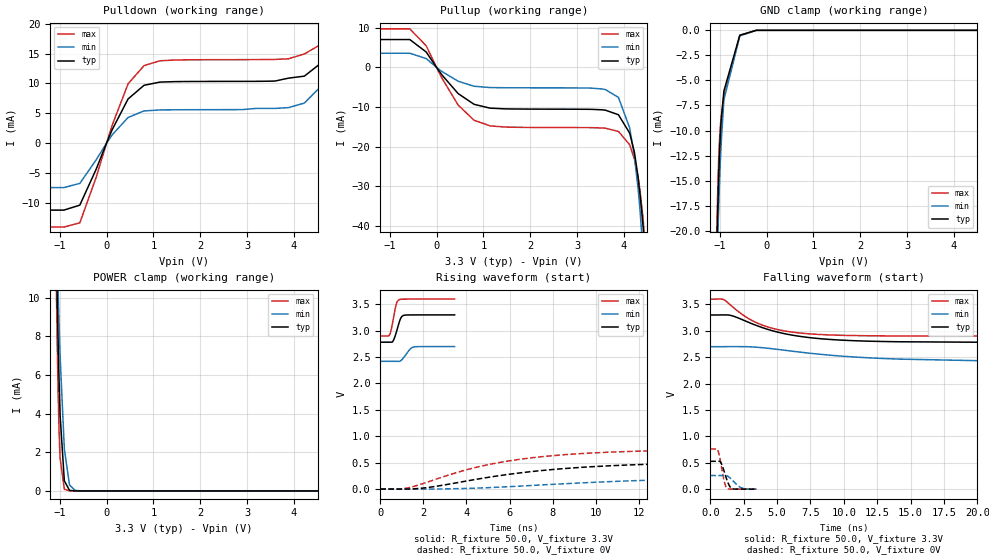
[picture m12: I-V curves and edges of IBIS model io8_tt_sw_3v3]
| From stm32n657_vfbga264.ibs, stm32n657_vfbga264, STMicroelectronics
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[Model]   io8_tt_sw_3v3
Model_type I/O
Polarity   Non-Inverting
Enable   Active-Low
| CAP_THRESHOLD on pad IOTT is "UDTCAPC" :
| Rising=30.0% of vddiov33sw   Falling=70.0% of vddiov33sw
| C_comp min and max val. don't necessarily correlate with the min and max pvt
| but are the smallest and greatest pad capacitance found.
| var   typ   min   max
C_comp   1.00484pF  998.37000fF  1.02526pF
|C_comp_pullup   499.19000fF  510.35000fF  493.55000fF
|C_comp_pulldown   505.65000fF  488.02000fF  531.70936fF
Vinl = 810.0mV
Vinh = 2.52V
Vmeas = 1.65V   | Reference voltage for timing measurements
Cref  = 50.0pF   | Timing specification test load capacitance value
Rref  = 100.0MOhm   | Timing specification test load resistance value
Vref  = 1.65V   | Timing specification test load voltage
[Model Spec]
| TIME_THRESHOLD on pin ZIV08SW is "CMOS" :
| Rising=50.0% of vddv08sw   Falling=50.0% of vddv08sw
Vinl 1.08570V 868.70000mV 1.21270V
Vinh 1.55630V 1.26330V 1.71030V
| variable   typ   min   max
[Temperature Range] 25.0 125.0 -40.0
| variable   typ   min   max
[Voltage Range] 3.3V 2.7V 3.6V
| variable   typ   min   max
[POWER Clamp Reference] 3.3V 2.7V 3.6V
| variable   typ   min   max
[GND Clamp Reference] 0V 0V 0V
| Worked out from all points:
|   slope of the pulldown table from 0 to 0.495 V, typ, clamps not added: 64.8 ohm
|   slope of the pullup table from 0 to 0.495 V, typ, clamps not added: 71.9 ohm
|   POWER clamp passes 1 mA (typ) near -0.91 V on its own axis
|   rising waveform, R_fixture 50.0, V_fixture 3.3V: 20-80 % time 231ps typ, 315ps min, 198ps max; typ from 2.78 V to 3.3 V
|   falling waveform, R_fixture 50.0, V_fixture 3.3V: 20-80 % time 4.43ns typ, 7.79ns min, 3.12ns max; typ from 3.3 V to 2.78 V
|   rising waveform, R_fixture 50.0, V_fixture 0V: 20-80 % time 6.45ns typ, 10.5ns min, 5.05ns max; typ from 0 V to 0.528 V
|   falling waveform, R_fixture 50.0, V_fixture 0V: 20-80 % time 423ps typ, 646ps min, 342ps max; typ from 0.528 V to 0 V
[POWER Clamp]
-3.3V     1.206A     322.9mA    1.949A
-1.07V    12.25mA    13.82mA    10.53mA
-1.06V    10.95mA    12.86mA    8.87mA
-1.05V    9.71mA     11.93mA    7.356mA
-1.03V    7.448mA    10.14mA    4.814mA
-1.02V    6.433mA    9.297mA    3.795mA
-1V       4.655mA    7.705mA    2.244mA
-990mV    3.898mA    6.963mA    1.687mA
-900mV    522uA      2.17mA     91.57uA
-790mV    29.02uA    304.6uA    2.409uA
-670mV    1.227uA    28.29uA    197.5nA
6.6V      0A         0A         0A
[GND Clamp]
-3.3V     -3.522A    -2.678A    -3.669A
-1.06V    -21.86mA   -24.42mA   -19.94mA
-1.05V    -19.75mA   -22.51mA   -17.72mA
-1.04V    -17.84mA   -20.74mA   -15.8mA
-1.03V    -16.13mA   -19.1mA    -14.17mA
-1.01V    -13.21mA   -16.17mA   -11.65mA
-980mV    -9.97mA    -12.54mA   -9.281mA
-970mV    -9.148mA   -11.51mA   -8.745mA
-910mV    -6.061mA   -6.933mA   -6.693mA
-570mV    -485.4uA   -556.9uA   -511.9uA
-220mV    -47.03nA   -390.1nA   -38.88nA
6.6V      80.36nA    707.4nA    100.1nA
| variable   typ   min   max
[Pullup Reference] 3.3V 2.7V 3.6V
| variable   typ   min   max
[Pulldown Reference] 0V 0V 0V
[Pullup]
-3.3V     7.046mA    3.582mA    9.739mA
-570mV    7.046mA    3.582mA    9.739mA
-220mV    3.9mA      2.233mA    5.468mA
460mV     -6.603mA   -3.484mA   -9.498mA
800mV     -9.321mA   -4.753mA   -13.34mA
3.6V      -10.79mA   -5.593mA   -15.36mA
3.88V     -11.95mA   -7.582mA   -16.17mA
4.12V     -16.61mA   -15.29mA   -19.54mA
4.3V      -27.8mA    -30.71mA   -27.83mA
4.4V      -39.38mA   -45.7mA    -37.53mA
4.42V     -42.33mA   -49.4mA    -40.43mA
6.6V      -162.2mA   -862.2mA   -164.4mA
[Pulldown]
-3.3V     -11.22mA   -7.442mA   -14.05mA
-910mV    -11.22mA   -7.442mA   -14.05mA
-570mV    -10.38mA   -6.74mA    -13.35mA
120mV     2.252mA    1.384mA    2.997mA
460mV     7.403mA    4.305mA    9.944mA
800mV     9.692mA    5.397mA    12.98mA
3.6V      10.41mA    5.82mA     14.02mA
4.22V     11.22mA    6.712mA    14.93mA
4.56V     13.32mA    9.4mA      16.49mA
4.9V      20.4mA     17.95mA    22.55mA
5.23V     40.75mA    40.8mA     40.72mA
6.6V      253mA      251.5mA    251.6mA
[Ramp]
dV/dt_r 316.76689mV/6.44533ns 154.93407mV/10.06847ns 455.99238mV/5.04952ns
dV/dt_f 310.42989mV/4.42676ns 168.29468mV/7.79063ns 419.63652mV/3.11752ns
R_load = 50.0
| Removed startup time: 0s 0s 0s  .
| Removed end time: 3.45ns.
[Rising Waveform]
R_fixture   = 50.0
V_fixture   = 3.3V
V_fixture_min = 2.7V
V_fixture_max = 3.6V
0s        2.783V     2.42V      2.901V
400ps     2.783V     2.42V      2.9V
450ps     2.783V     2.42V      2.937V
600ps     2.808V     2.42V      3.211V
750ps     2.978V     2.42V      3.518V
850ps     3.121V     2.419V     3.582V
950ps     3.239V     2.432V     3.595V
1.05ns    3.285V     2.473V     3.598V
1.55ns    3.299V     2.691V     3.599V
3.45ns    3.3V       2.7V       3.6V
| Removed startup time: 0s 0s 0s  .
| Removed end time: 59.9ns.
[Falling Waveform]
R_fixture   = 50.0
V_fixture   = 3.3V
V_fixture_min = 2.7V
V_fixture_max = 3.6V
0s        3.3V       2.7V       3.6V
1ns       3.301V     2.7V       3.59V
1.6ns     3.288V     2.701V     3.47V
2.7ns     3.179V     2.7V       3.258V
4.2ns     3.036V     2.673V     3.081V
5.9ns     2.929V     2.622V     2.984V
8.4ns     2.848V     2.551V     2.928V
13.3ns    2.796V     2.472V     2.904V
20ns      2.784V     2.435V     2.901V
59.9ns    2.783V     2.42V      2.901V
| Removed startup time: 0s 0s 0s  .
| Removed end time: 69.9ns.
[Rising Waveform]
R_fixture   = 50.0
V_fixture   = 0V
V_fixture_min = 0V
V_fixture_max = 0V
0s        488.3nV    1.411uV    485.2nV
900ps     -2.101mV   -677.2uV   -502.8uV
1.3ns     27.55uV    -1.128mV   23.84mV
2.3ns     34.32mV    56uV       146.8mV
4.1ns     158.7mV    12.61mV    375.1mV
6.2ns     290.9mV    49.36mV    547.3mV
8.6ns     389.5mV    101.2mV    651.9mV
12ns      462.6mV    160.8mV    717.5mV
23.3ns    521.7mV    238.4mV    757.9mV
69.9ns    527.9mV    258.2mV    760mV
| Removed startup time: 0s 0s 0s  .
| Removed end time: 3.45ns.
[Falling Waveform]
R_fixture   = 50.0
V_fixture   = 0V
V_fixture_min = 0V
V_fixture_max = 0V
0s        527.9mV    258.3mV    760mV
550ps     527.9mV    258.3mV    750.2mV
650ps     528.1mV    258.3mV    666.3mV
800ps     499.6mV    258.3mV    475.2mV
1.05ns    329.3mV    258.2mV    142.7mV
1.25ns    171.3mV    253.9mV    15.73mV
1.45ns    56.19mV    218.7mV    1.746mV
1.65ns    9.27mV     171.4mV    790uV
2.35ns    435uV      23.87mV    281.2uV
3.45ns    165.1uV    363.5uV    128uV
